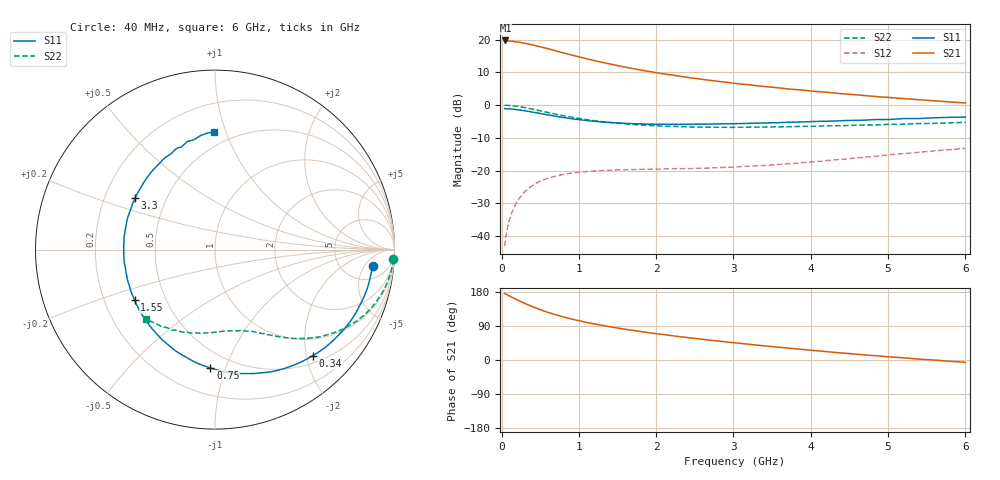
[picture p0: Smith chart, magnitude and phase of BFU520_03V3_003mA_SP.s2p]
! Filename:  P:\Prog\Test\Noise\ATS_data\Testdata_Net\03 Spar\BFU520_APG2013_37_A05_03p3V_003mA_SP_CM01_D.s2p
! Date/Time: Fri 26/Apr/2013 13:00:02
! BFU520_APG2013_37_A05_03p3V_1to20mA_SP_CM01_Bias3_R.s2p
! MDIF S-parameter v. bias file
! BFU520_APG2013_37_A05_03p3V_1to20mA_SP_CM01
! Date/time Tue Apr 23 14:11:50 2013
! VAR V_out= 3.3000
! VAR I_out= 3.0000
! VAR V_in= 0.8187
! VAR I_in= 0.0342
! Device data file deembeded for feedlines and parallel
! Original file: \03 Spar\BFU520_APG2013_37_A05_03p3V_003mA_SP_CM01_R.s2p
! Feed-files: PR047V01_250413_Feed1.s2p, PR047V01_250413_Feed2.s2p
! Parallel-file: PR047V01_250413_Par.s2p
# MHz S MA R 50
!  Freq-MHz  S11-mag  S11-arg  S21-mag  S21-arg  S12-mag  S12-arg  S22-mag  S22-arg
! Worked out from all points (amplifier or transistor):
!   98 points, 40 MHz to 6 GHz, reference 50 ohm
!   highest |S21| = 19.7 dB at 50 MHz (marker M1)
!   |S21| within 3 dB of that: start of sweep to 674 MHz
!   unconditionally stable (mu >= 1): 2.666 GHz to 4.891 GHz
!   at 300 MHz: K = 0.14, MSG = 22.7 dB, |S12| = -26.5 dB
!   at 1.6 GHz: K = 0.66, MSG = 15.7 dB, |S12| = -19.7 dB
!   at 6 GHz: K = 0.86, MSG = 6.9 dB, |S12| = -13.2 dB
!   S11 on the Smith chart (normalised r, x): 40 MHz: 10, -8; 340 MHz: 0.64, -2.13; 750 MHz: 0.38, -0.89; 1.55 GHz: 0.33, -0.26; 3.3 GHz: 0.33, +0.26; 6 GHz: 0.40, +0.91
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40  0.8832 -5.9  9.684 175.8  0.006996 86.4  0.9945 -3.1
50  0.8813 -7.3  9.71 174.1  0.008645 85.4  0.9936 -3.9
60  0.8799 -8.5  9.578 173.4  0.01042 84.8  0.9933 -4.8
70  0.8786 -10.0  9.595 172.6  0.0121 84.0  0.9909 -5.6
120  0.871 -17.4  9.528 167.0  0.02052 80.0  0.9808 -9.5
220  0.8454 -31.4  9.169 157.0  0.03617 72.0  0.9485 -17.1
340  0.8043 -47.3  8.613 145.9  0.05213 63.5  0.8957 -25.1
440  0.7674 -59.6  8.088 137.5  0.06308 57.5  0.8476 -30.9
550  0.7242 -72.4  7.525 129.2  0.0724 51.6  0.7929 -36.4
600  0.7073 -77.7  7.275 125.8  0.0762 49.4  0.7712 -38.6
750  0.6603 -92.3  6.497 116.5  0.08485 43.6  0.7091 -44.3
900  0.6196 -105.4  5.85 108.5  0.09108 39.2  0.6571 -48.9
1050  0.5892 -117.0  5.278 101.4  0.09515 35.7  0.6126 -52.8
1300  0.5523 -133.6  4.504 91.4  0.09989 31.7  0.5591 -58.0
1550  0.5294 -147.8  3.904 82.8  0.1027 29.1  0.5223 -62.5
2050  0.5103 -170.7  3.058 68.2  0.1053 27.4  0.4789 -70.6
2450  0.5098 173.6  2.604 58.1  0.1073 28.0  0.4629 -77.0
3100  0.5223 153.0  2.097 43.6  0.1144 31.8  0.4583 -86.8
3300  0.5295 147.3  1.979 39.4  0.1178 33.0  0.4604 -90.1
4100  0.5638 127.1  1.603 24.0  0.138 37.2  0.476 -103.0
5200  0.6221 104.3  1.256 5.8  0.1815 37.6  0.5102 -121.4
6000  0.655 90.7  1.079 -6.2  0.2188 34.0  0.5437 -135.1
